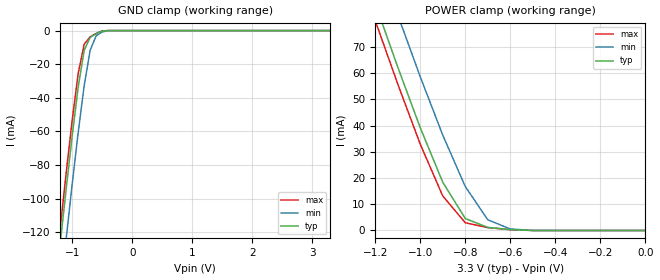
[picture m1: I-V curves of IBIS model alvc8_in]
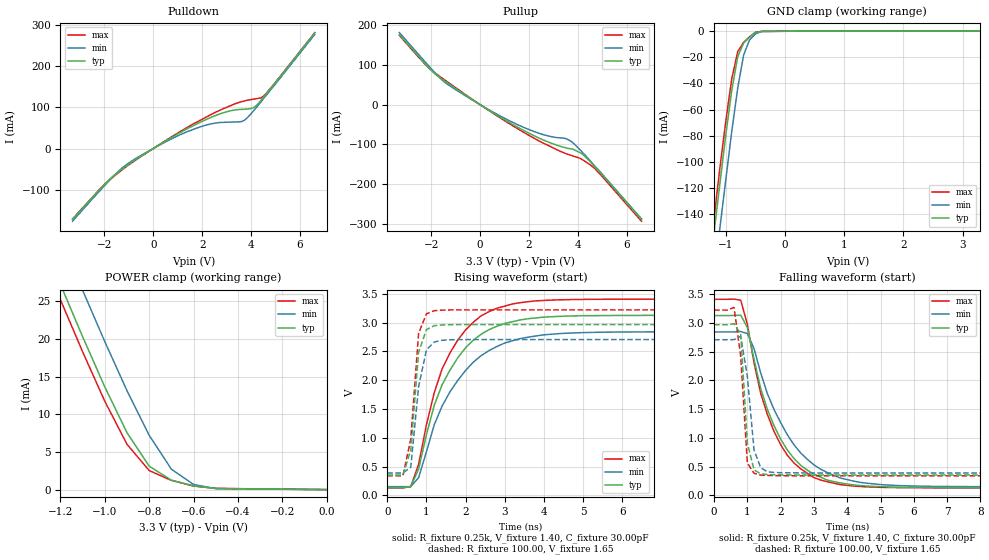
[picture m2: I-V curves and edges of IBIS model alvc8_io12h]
| IBIS file 62245ahr.ibs created by s2ibis2 version 1.1
| North Carolina State University Electronics Research Laboratory  1995
[IBIS ver]   2.1
[File name]   62245ahr.ibs
[File Rev]   1.0
[Date]   03/01/99 rtk rtk
[Source]   Integrated Device Technology, Inc.
[Notes]   1.Temperatures: typ=25C, min=100C, max=0C 2.RRmp rates based
   on 50 ohm load.
[Disclaimer] Integrated Device Technology, Inc. ("IDT") hereby grants the
   user of this IBIS model a non-exclusive, nontransferable
   license to use this IBIS model under the following terms. The
   user is granted this license only to use the IBIS model and is
   not granted rights to sell, copy (except as needed to run the
   IBIS model), rent, lease or sub-license the IBIS model in
   whole or in part, or in modified form to anyone. The User may
   modify the IBIS model to suit its specific applications, but
   rights to derivative works and such modifications shall belong
   to IDT. This IBIS model is provided on an AS IS" basis and IDT
   makes absolutely no warranty with respect to the information
   contained herein. IDT DISCLAIMS AND CUSTOMER WAIVES ALL
   WARRANTIES, EXPRESS AND IMPLIED, INCLUDING WARRANTIES OF
   MERCHANTABILITY AND FITNESS FOR A PARTICULAR PURPOSE. THE
   ENTIRE RISK AS TO QUALITY AND PERFORMANCE IS WITH THE USER
   ACCORDINGLY, IN NO EVENT SHALL IDT BE LIABLE FOR ANY DIRECT OR
   INDIRECT DAMAGES, WHETHER IN CONTRACT OR TORT, INCLUDING ANY
   LOST PROFITS OR OTHER INCIDENTAL, CONSEQUENTIAL, EXEMPLARY, OR
   PUNITIVE DAMAGES ARISING OUT OF THE USE OR APPLICATION OF THE
   IBIS model. Further, IDT reserves the right to make changes
   without notice to any product herein to improve reliability,
   function, or design. IDT does not convey any license under
   patent rights or any other intellectual property rights,
   including those of third parties. IDT is not obligated to
   provide maintenance or support for the licensed IBIS model.
[Copyright]   Copyright 1997, Integrated Device Technology, Inc. all rights
   reserved
|   Component ALVCHR162245
[Component]   ALVCHR162245
[Manufacturer]   Integrated Device Technology
[Package]
| PA48
| variable   typ   min   max
R_pkg   6.50m   5.00m   10.00m
L_pkg   3.20nH   2.50nH   4.40nH
C_pkg   0.27pF   0.01pF   0.98pF
| PV48   typ   min   max
|R_pkg   6.5m   5.00m   10.00m
|L_pkg   4.75nH   3.82nH   6.72nH
|C_pkg   0.24pF   0.01pF   1.55pF
[Pin]  signal_name   model_name   R_pin   L_pin   C_pin
1   1DIR   alvc8_in
2   1B1   alvc8_io12h
3   1B2   alvc8_io12h
4   GND   GND
5   1B3   alvc8_io12h
6   1B4   alvc8_io12h
7   VCC   POWER
8   1B5   alvc8_io12h
9   1B6   alvc8_io12h
10   GND   GND
11   1B7   alvc8_io12h
12   1B8   alvc8_io12h
13   2B1   alvc8_io12h
14   2B2   alvc8_io12h
15   GND   GND
16   2B3   alvc8_io12h
17   2B4   alvc8_io12h
18   VCC   POWER
19   2B5   alvc8_io12h
20   2B6   alvc8_io12h
21   GND   GND
22   2B7   alvc8_io12h
23   2B8   alvc8_io12h
24   2DIR   alvc8_in
25   2OEB   alvc8_in
26   2A8   alvc8_io12h
27   2A7   alvc8_io12h
28   GND   GND
29   2A6   alvc8_io12h
30   2A5   alvc8_io12h
31   VCC   POWER
32   2A4   alvc8_io12h
33   2A3   alvc8_io12h
34   GND   GND
35   2A2   alvc8_io12h
36   2A1   alvc8_io12h
37   1A8   alvc8_io12h
38   1A7   alvc8_io12h
39   GND   GND
40   1A6   alvc8_io12h
41   1A5   alvc8_io12h
42   VCC   POWER
43   1A4   alvc8_io12h
44   1A3   alvc8_io12h
45   GND   GND
46   1A2   alvc8_io12h
47   1A1   alvc8_io12h
48   1OEB   alvc8_in
| Models and submodels in the file (2): alvc8_in (Input), alvc8_io12h (I/O)
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| in   in   dummy_model
| oe   oe   dummy_model
|   Model alvc8_in
[Model]   alvc8_in
Model_type   Input
Vinl =  0.800V
Vinh =  2.000V
C_comp   3.00pF   NA   NA
[Temperature Range]   25.00   100.00   0.000
[Voltage Range]   3.30V   3.00V   3.60V
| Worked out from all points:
|   GND clamp passes 1 mA (typ) near -0.54 V on its own axis
|   POWER clamp passes 1 mA (typ) near -0.68 V on its own axis
[GND_clamp]
| voltage   I(typ)   I(min)   I(max)
-3.3V     -860mA     -887mA     -851mA
-1.3V     -161mA     -190mA     -151mA
-1.2V     -127mA     -157mA     -118mA
-1.1V     -94.41mA   -124mA     -84.85mA
-1V       -62.78mA   -91.54mA   -53.52mA
-900mV    -33.71mA   -60.78mA   -25.6mA
-800mV    -11.74mA   -32.83mA   -8.09mA
-700mV    -4.033mA   -11.65mA   -3.7mA
-600mV    -1.899mA   -3.108mA   -1.699mA
-500mV    -308uA     -810uA     -172uA
-400mV    -3.848nA   -9.872uA   -399pA
3.3V      39.6pA     19.33nA    26.4pA
[POWER_clamp]
| voltage   I(typ)   I(min)   I(max)
-3.3V     630mA      648mA      624mA
-1.2V     86.56mA    106mA      80.02mA
-1.1V     62.33mA    82.22mA    55.88mA
-1V       39.2mA     58.61mA    32.91mA
-900mV    18.4mA     36.35mA    13.15mA
-800mV    4.556mA    16.76mA    2.954mA
-700mV    1.164mA    4.056mA    1.087mA
-600mV    320uA      578uA      299uA
-500mV    40.08nA    12.23uA    3.465nA
0V        39.6pA     59.11pA    43.2pA
|   Model alvc8_io12h
[Model]   alvc8_io12h
Model_type   I/O
Polarity   Non-Inverting
Enable   Active-High
Vinl =  0.000V
Vinh =  2.000V
Vmeas =  1.500V
C_comp   3.00pF   NA   NA
[Temperature Range]   25.00   100.00   0.000
[Voltage Range]   3.30V   3.00V   3.60V
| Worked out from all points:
|   slope of the pulldown table from 0 to 0.495 V, typ, clamps not added: 27.5 ohm
|   slope of the pullup table from 0 to 0.495 V, typ, clamps not added: 25.8 ohm
|   GND clamp passes 1 mA (typ) near -0.50 V on its own axis
|   POWER clamp passes 1 mA (typ) near -0.67 V on its own axis
|   rising waveform, R_fixture 0.25k, V_fixture 1.40, C_fixture 30.00pF: 20-80 % time 1.07ns typ, 1.21ns min, 991ps max; typ from 0.137 V to 3.12 V
|   rising waveform, R_fixture 100.00, V_fixture 1.65: 20-80 % time 184ps typ, 259ps min, 200ps max; typ from 0.354 V to 2.96 V
|   falling waveform, R_fixture 0.25k, V_fixture 1.40, C_fixture 30.00pF: 20-80 % time 1.13ns typ, 1.37ns min, 1.04ns max; typ from 3.12 V to 0.137 V
|   falling waveform, R_fixture 100.00, V_fixture 1.65: 20-80 % time 176ps typ, 241ps min, 216ps max; typ from 2.96 V to 0.354 V
[Pulldown]
| voltage   I(typ)   I(min)   I(max)
-3.3V     -172mA     -177mA     -171mA
-1.8V     -76mA      -78.1mA    -76.9mA
-1.3V     -51.4mA    -48.7mA    -53mA
-700mV    -26.3mA    -23.6mA    -27.4mA
800mV     28.7mA     25.1mA     30.3mA
1.8V      60.3mA     50.2mA     64.7mA
2.9V      87.5mA     63.7mA     97.9mA
3.7V      95.5mA     67.7mA     115mA
4.1V      99.3mA     91.8mA     120mA
4.5V      124mA      121mA      127mA
5V        161mA      157mA      161mA
6.6V      281mA      277mA      282mA
[Pullup]
| voltage   I(typ)   I(min)   I(max)
-3.3V     176mA      181mA      174mA
-1.9V     80.3mA     83.6mA     82mA
-1.5V     61.8mA     58.9mA     64.3mA
-1V       40.8mA     37.7mA     42.5mA
400mV     -15.6mA    -14.2mA    -16.4mA
1.7V      -62.2mA    -54.9mA    -66.6mA
2.9V      -96.6mA    -80.2mA    -106mA
3.5V      -108mA     -85.3mA    -123mA
3.8V      -112mA     -96mA      -129mA
4.2V      -125mA     -121mA     -139mA
4.7V      -156mA     -155mA     -161mA
6.6V      -289mA     -287mA     -293mA
[GND_clamp]
| voltage   I(typ)   I(min)   I(max)
-3.3V     -1.019A    -1.052A    -1.008A
-1.3V     -194mA     -229mA     -182mA
-1.2V     -154mA     -189mA     -143mA
-1.1V     -116mA     -150mA     -104mA
-1V       -78.66mA   -113mA     -68.13mA
-900mV    -44.91mA   -76.33mA   -36.12mA
-800mV    -19.38mA   -43.36mA   -15.48mA
-700mV    -9.002mA   -18.09mA   -8.455mA
-600mV    -4.636mA   -6.615mA   -4.212mA
-500mV    -941uA     -2.052mA   -652uA
-400mV    -144uA     -128uA     -169uA
3.3V      264uA      161uA      341uA
[POWER_clamp]
| voltage   I(typ)   I(min)   I(max)
-3.3V     183mA      189mA      181mA
-1.3V     34.33mA    40.55mA    32.29mA
-1.2V     27.22mA    33.44mA    25.19mA
-1.1V     20.28mA    26.44mA    18.28mA
-1V       13.61mA    19.62mA    11.71mA
-900mV    7.542mA    13.11mA    6.005mA
-800mV    3.103mA    7.194mA    2.527mA
-700mV    1.249mA    2.702mA    1.219mA
-600mV    484uA      674uA      476uA
-500mV    146uA      134uA      162uA
0V        111pA      156pA      121pA
[Ramp]
| variable   typ   min   max
dV/dt_r   1.29/0.24n   1.13/0.30n   1.44/0.25n
dV/dt_f   1.26/0.26n   1.08/0.26n   1.40/0.24n
R_load = 50.00
[Rising Waveform]
R_fixture = 0.25k
V_fixture = 1.40
C_fixture = 30.00pF
R_dut = 7.00m
L_dut = 3.30nH
C_dut = 0.29pF
| time   V(typ)   V(min)   V(max)
0s        137mV      152mV      131mV
600ps     152mV      153mV      153mV
800ps     459mV      307mV      538mV
1.2ns     1.566V     1.227V     1.783V
1.4ns     1.921V     1.551V     2.196V
1.8ns     2.389V     1.996V     2.696V
2.4ns     2.799V     2.427V     3.119V
3.2ns     3.016V     2.685V     3.324V
5.6ns     3.122V     2.834V     3.405V
19.8ns    3.125V     2.84V      3.407V
[Rising Waveform]
R_fixture = 100.00
V_fixture = 1.65
R_dut = 7.00m
L_dut = 3.30nH
C_dut = 0.29pF
| time   V(typ)   V(min)   V(max)
0s        354mV      389mV      341mV
400ps     354mV      390mV      341mV
600ps     788mV      488mV      976mV
800ps     2.487V     1.886V     2.814V
1ns       2.877V     2.527V     3.153V
1.2ns     2.947V     2.663V     3.206V
1.4ns     2.959V     2.693V     3.216V
2ns       2.965V     2.705V     3.22V
19.8ns    2.965V     2.705V     3.22V
[Falling Waveform]
R_fixture = 0.25k
V_fixture = 1.40
C_fixture = 30.00pF
R_dut = 7.00m
L_dut = 3.30nH
C_dut = 0.29pF
| time   V(typ)   V(min)   V(max)
0s        3.125V     2.84V      3.407V
800ps     3.131V     2.846V     3.392V
1ns       2.917V     2.813V     2.972V
1.4ns     1.855V     2.128V     1.774V
1.8ns     1.213V     1.493V     1.113V
2.4ns     640mV      880mV      563mV
3.2ns     318mV      456mV      267mV
4.2ns     181mV      247mV      162mV
5.6ns     143mV      169mV      135mV
19.8ns    137mV      152mV      131mV
[Falling Waveform]
R_fixture = 100.00
V_fixture = 1.65
R_dut = 7.00m
L_dut = 3.30nH
C_dut = 0.29pF
| time   V(typ)   V(min)   V(max)
0s        2.965V     2.705V     3.22V
400ps     2.965V     2.705V     3.22V
600ps     2.984V     2.706V     3.266V
800ps     2.805V     2.763V     2.411V
1ns       908mV      2.064V     561mV
1.2ns     444mV      789mV      384mV
1.4ns     374mV      481mV      353mV
1.6ns     362mV      411mV      347mV
2ns       357mV      394mV      343mV
19.8ns    354mV      389mV      341mV
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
